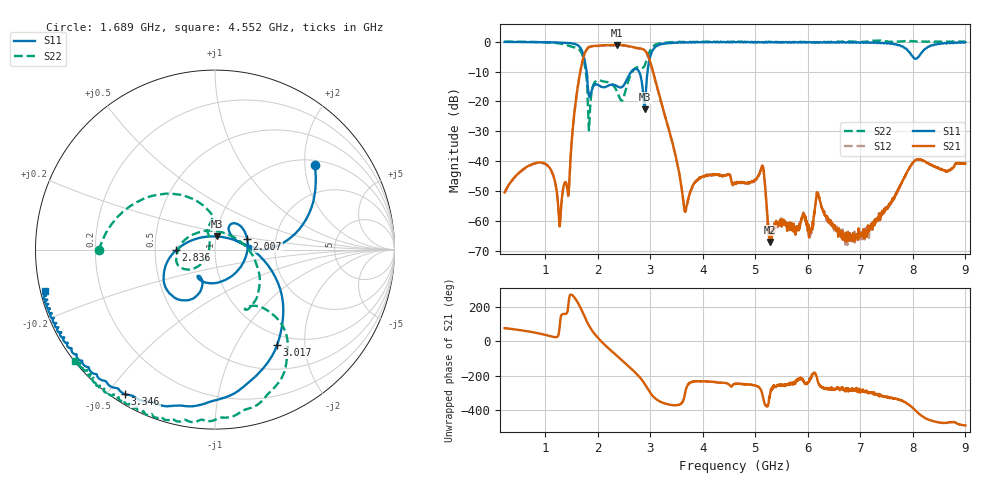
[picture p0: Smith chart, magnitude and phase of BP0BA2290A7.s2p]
!Agilent Technologies,E8358A,US41080443,A.07.50.56
!Agilent E8358A: A.07.50.56
!Date: Thursday, November 09, 2017 08:42:52
!Correction: S11(Full 2 Port(1,2))
!S21(Full 2 Port(1,2))
!S12(Full 2 Port(1,2))
!S22(Full 2 Port(1,2))
!S2P File: Measurements: S11, S21, S12, S22:
# Hz S  dB  R 50
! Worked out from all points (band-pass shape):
!   1601 points, 225 MHz to 9 GHz, reference 50 ohm
!   highest |S21| = -1.11 dB at 2.369 GHz (marker M1); lowest = -67.0 dB at 5.276 GHz (marker M2)
!   |S21| within 3 dB of the highest: 1.746 GHz to 2.941 GHz (1.195 GHz wide, 51 % of centre)
!   lowest |S11| = -22.6 dB at 2.89 GHz (marker M3), VSWR 1.16, Z = 50.5 + j7.43 ohm
!   |S11| at or under -10 dB: 1.786 GHz to 2.639 GHz (853.1 MHz wide, 38.6 % of centre); 2.783 GHz to 2.946 GHz (163.1 MHz wide, 5.69 % of centre)
!   |S22| runs from -29.7 to 0.4 dB; largest |S21 - S12| = 0.017
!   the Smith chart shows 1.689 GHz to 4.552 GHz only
!   S11 on the Smith chart (normalised r, x): 1.689 GHz: 1.11, +2.24; 2.007 GHz: 1.42, +0.18; 2.836 GHz: 0.64, -0.00; 3.017 GHz: 0.84, -1.50; 3.346 GHz: 0.03, -0.56; 4.552 GHz: 0.01, -0.12
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2.25e8  -0.08 172.3  -50.42 76.8  -50.56 77.2  0.02 169.0
9.70875e8  -0.18 142.0  -40.59 39.8  -40.75 39.9  -0.19 118.4
1.283484e9  -0.29 121.0  -60.15 122.8  -60.33 122.7  -0.64 63.4
1.552219e9  -0.71 84.0  -24.03 -104.2  -24.22 -103.8  -1.93 -73.2
1.689328e9  -2.74 40.4  -7.93 -176.0  -8.04 -175.6  -3.78 -179.6
2.007422e9  -14.48 18.3  -1.33 18.6  -1.48 18.8  -12.95 -161.4
2.369391e9  -14.94 -123.1  -1.11 -85.0  -1.27 -84.9  -16.87 142.3
2.835562e9  -13.28 -179.1  -2.36 138.0  -2.48 138.1  -8.67 -62.5
2.890406e9  -22.63 81.8  -2.84 113.9  -2.98 114.0  -8.02 -52.8
3.016547e9  -3.96 -56.9  -7.87 53.4  -8.03 53.5  -2.31 -59.2
3.153656e9  -1.13 -97.3  -16.83 15.7  -16.99 16.0  -0.64 -82.8
3.345609e9  -0.46 -121.9  -28.88 -6.1  -29.07 -5.8  -0.24 -100.8
3.669188e9  -0.21 -141.0  -55.90 66.4  -56.70 67.6  -0.12 -116.6
4.552172e9  -0.23 -166.2  -46.96 98.8  -47.27 100.3  -0.02 -141.3
4.6125e9  -0.16 -167.8  -47.11 113.8  -47.50 112.9  0.02 -142.7
5.128031e9  -0.17 -179.9  -41.47 59.4  -41.65 59.6  -0.13 -156.0
5.276109e9  -0.24 176.9  -67.02 45.2  -65.71 38.0  -0.04 -160.8
6.076828e9  -0.28 156.2  -62.02 162.4  -62.77 163.3  -0.21 175.8
7.541156e9  -0.49 106.2  -54.43 32.7  -55.03 34.2  -0.05 142.6
7.963453e9  -4.28 19.1  -41.40 -17.5  -41.45 -17.6  0.22 136.9
8.138953e9  -4.32 -104.7  -39.41 -66.0  -39.49 -66.0  -0.02 136.6
9e9  -0.18 150.8  -40.70 -128.7  -40.84 -127.8  -0.01 131.8
